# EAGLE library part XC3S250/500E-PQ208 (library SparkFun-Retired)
Xilinx Spartan3E FPGA Not in catalog
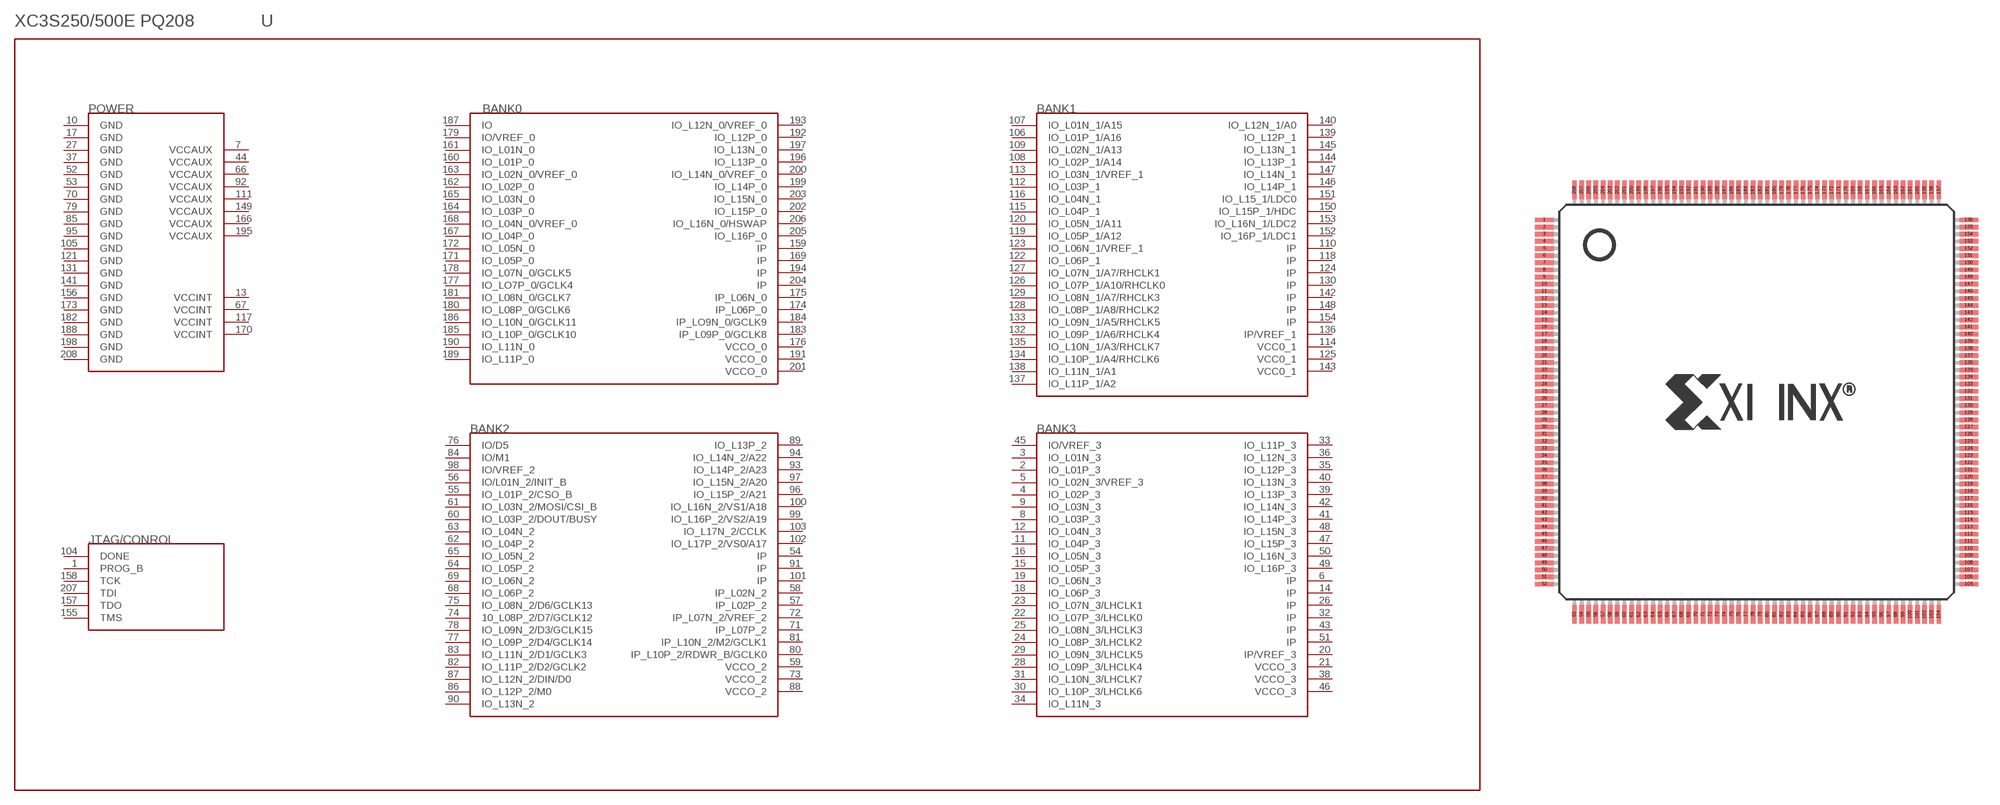
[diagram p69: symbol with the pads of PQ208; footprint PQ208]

Designator prefix -

## XC3S250/500E-PQ208  [PQ208]
1  PROG_B
2  IO_L01P_3
3  IO_L01N_3
4  IO_L02P_3
5  IO_L02N_3/VREF_3
6  IP
7  VCCAUX
8  IO_L03P_3
9  IO_L03N_3
10  GND
11  IO_L04P_3
12  IO_L04N_3
13  VCCINT
14  IP
15  IO_L05P_3
16  IO_L05N_3
17  GND
18  IO_L06P_3
19  IO_L06N_3
20  IP/VREF_3
21  VCCO_3
22  IO_L07P_3/LHCLK0
23  IO_L07N_3/LHCLK1
24  IO_L08P_3/LHCLK2
25  IO_L08N_3/LHCLK3
26  IP
27  GND
28  IO_L09P_3/LHCLK4
29  IO_L09N_3/LHCLK5
30  IO_L10P_3/LHCLK6
31  IO_L10N_3/LHCLK7
32  IP
33  IO_L11P_3
34  IO_L11N_3
35  IO_L12P_3
36  IO_L12N_3
37  GND
38  VCCO_3
39  IO_L13P_3
40  IO_L13N_3
41  IO_L14P_3
42  IO_L14N_3
43  IP
44  VCCAUX
45  IO/VREF_3
46  VCCO_3
47  IO_L15P_3
48  IO_L15N_3
49  IO_L16P_3
50  IO_L16N_3
51  IP
52  GND
53  GND
54  IP
55  IO_L01P_2/CSO_B
56  IO/L01N_2/INIT_B
57  IP_L02P_2
58  IP_L02N_2
59  VCCO_2
60  IO_L03P_2/DOUT/BUSY
61  IO_L03N_2/MOSI/CSI_B
62  IO_L04P_2
63  IO_L04N_2
64  IO_L05P_2
65  IO_L05N_2
66  VCCAUX
67  VCCINT
68  IO_L06P_2
69  IO_L06N_2
70  GND
71  IP_L07P_2
72  IP_L07N_2/VREF_2
73  VCCO_2
74  10_L08P_2/D7/GCLK12
75  IO_L08N_2/D6/GCLK13
76  IO/D5
77  IO_L09P_2/D4/GCLK14
78  IO_L09N_2/D3/GCLK15
79  GND
80  IP_L10P_2/RDWR_B/GCLK0
81  IP_L10N_2/M2/GCLK1
82  IO_L11P_2/D2/GCLK2
83  IO_L11N_2/D1/GCLK3
84  IO/M1
85  GND
86  IO_L12P_2/M0
87  IO_L12N_2/DIN/D0
88  VCCO_2
89  IO_L13P_2
90  IO_L13N_2
91  IP
92  VCCAUX
93  IO_L14P_2/A23
94  IO_L14N_2/A22
95  GND
96  IO_L15P_2/A21
97  IO_L15N_2/A20
98  IO/VREF_2
99  IO_L16P_2/VS2/A19
100  IO_L16N_2/VS1/A18
101  IP
102  IO_L17P_2/VS0/A17
103  IO_L17N_2/CCLK
104  DONE
105  GND
106  IO_L01P_1/A16
107  IO_L01N_1/A15
108  IO_L02P_1/A14
109  IO_L02N_1/A13
110  IP
111  VCCAUX
112  IO_L03P_1
113  IO_L03N_1/VREF_1
114  VCC0_1
115  IO_L04P_1
116  IO_L04N_1
117  VCCINT
118  IP
119  IO_L05P_1/A12
120  IO_L05N_1/A11
121  GND
122  IO_L06P_1
123  IO_L06N_1/VREF_1
124  IP
125  VCC0_1
126  IO_L07P_1/A10/RHCLK0
127  IO_L07N_1/A7/RHCLK1
128  IO_L08P_1/A8/RHCLK2
129  IO_L08N_1/A7/RHCLK3
130  IP
131  GND
132  IO_L09P_1/A6/RHCLK4
133  IO_L09N_1/A5/RHCLK5
134  IO_L10P_1/A4/RHCLK6
135  IO_L10N_1/A3/RHCLK7
136  IP/VREF_1
137  IO_L11P_1/A2
138  IO_L11N_1/A1
139  IO_L12P_1
140  IO_L12N_1/A0
141  GND
142  IP
143  VCC0_1
144  IO_L13P_1
145  IO_L13N_1
146  IO_L14P_1
147  IO_L14N_1
148  IP
149  VCCAUX
150  IO_L15P_1/HDC
151  IO_L15_1/LDC0
152  IO_16P_1/LDC1
153  IO_L16N_1/LDC2
154  IP
155  TMS
156  GND
157  TDO
158  TCK
159  IP
160  IO_L01P_0
161  IO_L01N_0
162  IO_L02P_0
163  IO_L02N_0/VREF_0
164  IO_L03P_0
165  IO_L03N_0
166  VCCAUX
167  IO_L04P_0
168  IO_L04N_0/VREF_0
169  IP
170  VCCINT
171  IO_L05P_0
172  IO_L05N_0
173  GND
174  IP_L06P_0
175  IP_L06N_0
176  VCCO_0
177  IO_LO7P_0/GCLK4
178  IO_L07N_0/GCLK5
179  IO/VREF_0
180  IO_L08P_0/GCLK6
181  IO_L08N_0/GCLK7
182  GND
183  IP_L09P_0/GCLK8
184  IP_LO9N_0/GCLK9
185  IO_L10P_0/GCLK10
186  IO_L10N_0/GCLK11
187  IO
188  GND
189  IO_L11P_0
190  IO_L11N_0
191  VCCO_0
192  IO_L12P_0
193  IO_L12N_0/VREF_0
194  IP
195  VCCAUX
196  IO_L13P_0
197  IO_L13N_0
198  GND
199  IO_L14P_0
200  IO_L14N_0/VREF_0
201  VCCO_0
202  IO_L15P_0
203  IO_L15N_0
204  IP
205  IO_L16P_0
206  IO_L16N_0/HSWAP
207  TDI
208  GND

## Footprint PQ208 (pad centres in mm)
smd 1.3 x 0.32: 1 -14.85,12.75; 2 -14.85,12.25; 3 -14.85,11.75; 4 -14.85,11.25; 5 -14.85,10.75; 6 -14.85,10.25; 7 -14.85,9.75; 8 -14.85,9.25; 9 -14.85,8.75; 10 -14.85,8.25; 11 -14.85,7.75; 12 -14.85,7.25; 13 -14.85,6.75; 14 -14.85,6.25; 15 -14.85,5.75; 16 -14.85,5.25; 17 -14.85,4.75; 18 -14.85,4.25; 19 -14.85,3.75; 20 -14.85,3.25; 21 -14.85,2.75; 22 -14.85,2.25; 23 -14.85,1.75; 24 -14.85,1.25; 25 -14.85,0.75; 26 -14.85,0.25; 27 -14.85,-0.25; 28 -14.85,-0.75; 29 -14.85,-1.25; 30 -14.85,-1.75; 31 -14.85,-2.25; 32 -14.85,-2.75; 33 -14.85,-3.25; 34 -14.85,-3.75; 35 -14.85,-4.25; 36 -14.85,-4.75; 37 -14.85,-5.25; 38 -14.85,-5.75; 39 -14.85,-6.25; 40 -14.85,-6.75; 41 -14.85,-7.25; 42 -14.85,-7.75; 43 -14.85,-8.25; 44 -14.85,-8.75; 45 -14.85,-9.25; 46 -14.85,-9.75; 47 -14.85,-10.25; 48 -14.85,-10.75; 49 -14.85,-11.25; 50 -14.85,-11.75; 51 -14.85,-12.25; 52 -14.85,-12.75; 105 14.85,-12.75; 106 14.85,-12.25; 107 14.85,-11.75; 108 14.85,-11.25; 109 14.85,-10.75; 110 14.85,-10.25; 111 14.85,-9.75; 112 14.85,-9.25; 113 14.85,-8.75; 114 14.85,-8.25; 115 14.85,-7.75; 116 14.85,-7.25; 117 14.85,-6.75; 118 14.85,-6.25; 119 14.85,-5.75; 120 14.85,-5.25; 121 14.85,-4.75; 122 14.85,-4.25; 123 14.85,-3.75; 124 14.85,-3.25; 125 14.85,-2.75; 126 14.85,-2.25; 127 14.85,-1.75; 128 14.85,-1.25; 129 14.85,-0.75; 130 14.85,-0.25; 131 14.85,0.25; 132 14.85,0.75; 133 14.85,1.25; 134 14.85,1.75; 135 14.85,2.25; 136 14.85,2.75; 137 14.85,3.25; 138 14.85,3.75; 139 14.85,4.25; 140 14.85,4.75; 141 14.85,5.25; 142 14.85,5.75; 143 14.85,6.25; 144 14.85,6.75; 145 14.85,7.25; 146 14.85,7.75; 147 14.85,8.25; 148 14.85,8.75; 149 14.85,9.25; 150 14.85,9.75; 151 14.85,10.25; 152 14.85,10.75; 153 14.85,11.25; 154 14.85,11.75; 155 14.85,12.25; 156 14.85,12.75
smd 0.32 x 1.3: 53 -12.75,-14.85; 54 -12.25,-14.85; 55 -11.75,-14.85; 56 -11.25,-14.85; 57 -10.75,-14.85; 58 -10.25,-14.85; 59 -9.75,-14.85; 60 -9.25,-14.85; 61 -8.75,-14.85; 62 -8.25,-14.85; 63 -7.75,-14.85; 64 -7.25,-14.85; 65 -6.75,-14.85; 66 -6.25,-14.85; 67 -5.75,-14.85; 68 -5.25,-14.85; 69 -4.75,-14.85; 70 -4.25,-14.85; 71 -3.75,-14.85; 72 -3.25,-14.85; 73 -2.75,-14.85; 74 -2.25,-14.85; 75 -1.75,-14.85; 76 -1.25,-14.85; 77 -0.75,-14.85; 78 -0.25,-14.85; 79 0.25,-14.85; 80 0.75,-14.85; 81 1.25,-14.85; 82 1.75,-14.85; 83 2.25,-14.85; 84 2.75,-14.85; 85 3.25,-14.85; 86 3.75,-14.85; 87 4.25,-14.85; 88 4.75,-14.85; 89 5.25,-14.85; 90 5.75,-14.85; 91 6.25,-14.85; 92 6.75,-14.85; 93 7.25,-14.85; 94 7.75,-14.85; 95 8.25,-14.85; 96 8.75,-14.85; 97 9.25,-14.85; 98 9.75,-14.85; 99 10.25,-14.85; 100 10.75,-14.85; 101 11.25,-14.85; 102 11.75,-14.85; 103 12.25,-14.85; 104 12.75,-14.85; 157 12.75,14.85; 158 12.25,14.85; 159 11.75,14.85; 160 11.25,14.85; 161 10.75,14.85; 162 10.25,14.85; 163 9.75,14.85; 164 9.25,14.85; 165 8.75,14.85; 166 8.25,14.85; 167 7.75,14.85; 168 7.25,14.85; 169 6.75,14.85; 170 6.25,14.85; 171 5.75,14.85; 172 5.25,14.85; 173 4.75,14.85; 174 4.25,14.85; 175 3.75,14.85; 176 3.25,14.85; 177 2.75,14.85; 178 2.25,14.85; 179 1.75,14.85; 180 1.25,14.85; 181 0.75,14.85; 182 0.25,14.85; 183 -0.25,14.85; 184 -0.75,14.85; 185 -1.25,14.85; 186 -1.75,14.85; 187 -2.25,14.85; 188 -2.75,14.85; 189 -3.25,14.85; 190 -3.75,14.85; 191 -4.25,14.85; 192 -4.75,14.85; 193 -5.25,14.85; 194 -5.75,14.85; 195 -6.25,14.85; 196 -6.75,14.85; 197 -7.25,14.85; 198 -7.75,14.85; 199 -8.25,14.85; 200 -8.75,14.85; 201 -9.25,14.85; 202 -9.75,14.85; 203 -10.25,14.85; 204 -10.75,14.85; 205 -11.25,14.85; 206 -11.75,14.85; 207 -12.25,14.85; 208 -12.75,14.85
